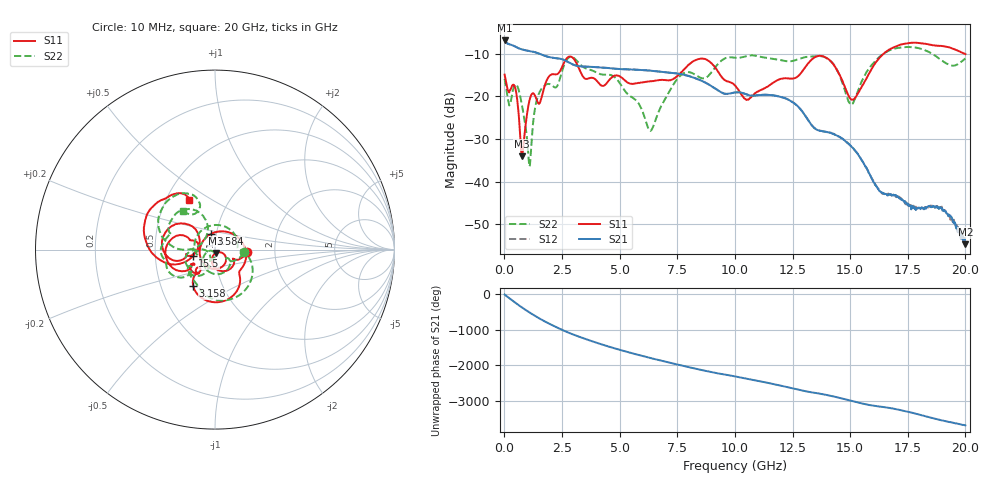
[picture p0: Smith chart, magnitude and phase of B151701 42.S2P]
!  2-Port S-parameters saved by WinCal
! VAR MeasName=S-Parameters (CALIBRATED_DATA) read from VNA (N5244A)
! VAR MeasDate=2015-12-24 19:14:22
! VAR NAME=B151701 42
! VAR FILENAME=B151701 42.S2P
! VAR DATE=2015-12-24 19:14:22
! VAR PHYS_PORTS=1,3
# Hz S DB R 50
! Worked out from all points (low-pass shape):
!   801 points, 10 MHz to 20 GHz, reference 50 ohm
!   highest |S21| = -6.89 dB at 10 MHz (marker M1); lowest = -54.7 dB at 20 GHz (marker M2)
!   |S21| within 3 dB of the highest: start of sweep to 1.46 GHz
!   lowest |S11| = -34.1 dB at 759.6 MHz (marker M3), VSWR 1.04, Z = 50.7 - j1.86 ohm
!   |S11| at or under -10 dB: start of sweep to 16.45 GHz; 19.97029 GHz to end of sweep
!   |S22| runs from -36.5 to -8.4 dB; largest |S21 - S12| = 0.00096
!   S11 on the Smith chart (normalised r, x): 10 MHz: 1.43, -0.04; 1.584 GHz: 0.94, +0.17; 3.158 GHz: 0.73, -0.31; 15.5 GHz: 0.78, -0.06; 20 GHz: 0.65, +0.40
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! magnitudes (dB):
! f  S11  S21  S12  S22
! 10 MHz  -14.9  -6.9  -6.9  -15.9
! 209.9 MHz  -19.1  -7.8  -7.8  -22.1
! 459.8 MHz  -17.9  -8.3  -8.3  -17.3
! 759.6 MHz  -34.1  -9.0  -9.0  -22.0
! 1.084 GHz  -21.1  -9.4  -9.4  -36.5
! 1.584 GHz  -20.8  -10.2  -10.2  -18.4
! 3.158 GHz  -12.5  -12.8  -12.9  -11.7
! 3.358 GHz  -14.9  -13.0  -13.0  -12.9
! 4.833 GHz  -15.1  -13.5  -13.5  -15.7
! 6.307 GHz  -16.5  -14.0  -14.0  -28.0
! 6.682 GHz  -16.2  -14.2  -14.2  -23.7
! 7.706 GHz  -14.2  -14.9  -14.9  -14.8
! 8.606 GHz  -11.1  -16.5  -16.5  -15.8
! 10.01 GHz  -17.5  -19.1  -19.1  -11.0
! 10.58 GHz  -20.8  -19.7  -19.7  -10.5
! 13.35 GHz  -11.3  -26.9  -26.9  -10.7
! 14.25 GHz  -12.3  -28.8  -28.8  -12.3
! 15.03 GHz  -20.7  -31.7  -31.7  -22.0
! 15.5 GHz  -17.8  -34.9  -35.0  -16.5
! 16.68 GHz  -9.1  -43.0  -42.9  -9.3
! 18.93 GHz  -8.1  -46.1  -46.0  -11.4
! 20 GHz  -10.1  -54.7  -55.2  -11.1
